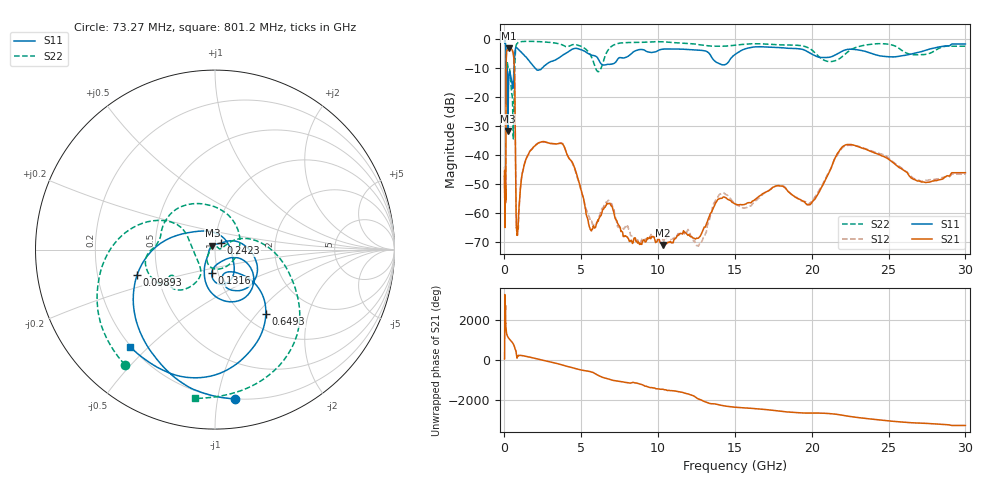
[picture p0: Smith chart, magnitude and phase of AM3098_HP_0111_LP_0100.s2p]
! Date/Time: Thu, Feb 28, 2019 8:38 AM
! Network Analyzer: Agilent Technologies E8364B Rev: A.07.50.67
! Sweep from 0.010 to 30.000 GHz, 1601 Points, Sweep Type: LOG
! Power Supply: 5.022 V, 0.002 A
# Hz S DB R 50
!freq MagS11 AngS11 MagS21 AngS21 MagS12 AngS12 MagS22 AngS22
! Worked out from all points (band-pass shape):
!   1601 points, 10 MHz to 30 GHz, reference 50 ohm
!   highest |S21| = -3.07 dB at 266.5 MHz (marker M1); lowest = -71.0 dB at 10.33 GHz (marker M2)
!   |S21| within 3 dB of the highest: 120.9 MHz to 602.1 MHz (481.2 MHz wide, 133 % of centre)
!   lowest |S11| = -31.6 dB at 232.8 MHz (marker M3), VSWR 1.05, Z = 48.5 + j2.13 ohm
!   |S11| at or under -10 dB: 102.2 MHz to 619.4 MHz (517.2 MHz wide, 143 % of centre); 2.012 GHz to 2.43 GHz (418.4 MHz wide, 18.8 % of centre)
!   |S22| runs from -34.3 to -0.5 dB; largest |S21 - S12| = 0.0098
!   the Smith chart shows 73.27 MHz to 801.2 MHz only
!   S11 on the Smith chart (normalised r, x): 73.27 MHz: 0.20, -1.12; 98.93 MHz: 0.38, -0.13; 131.6 MHz: 0.93, -0.25; 242.3 MHz: 1.07, +0.08; 649.3 MHz: 1.23, -1.12; 801.2 MHz: 0.20, -0.44
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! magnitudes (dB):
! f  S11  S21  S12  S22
! 10 MHz  -0.3  -47.1  -44.4  -0.5
! 38.04 MHz  -0.4  -59.5  -59.7  -0.8
! 73.27 MHz  -1.5  -54.0  -53.6  -1.8
! 86.86 MHz  -2.9  -51.9  -52.2  -3.0
! 98.93 MHz  -6.8  -26.3  -26.0  -7.8
! 131.6 MHz  -17.5  -4.9  -4.9  -10.3
! 144.7 MHz  -20.2  -4.1  -4.1  -11.2
! 184.9 MHz  -10.7  -3.7  -3.7  -8.0
! 232.8 MHz  -31.6  -3.2  -3.2  -9.7
! 242.3 MHz  -26.3  -3.2  -3.1  -9.8
! 266.5 MHz  -15.7  -3.1  -3.0  -10.1
! 550.5 MHz  -16.9  -4.4  -4.3  -30.3
! 649.3 MHz  -6.8  -10.8  -10.7  -14.3
! 801.2 MHz  -2.9  -65.9  -65.8  -1.5
! 2.084 GHz  -10.4  -36.3  -36.2  -0.7
! 3.798 GHz  -5.4  -36.2  -36.0  -2.0
! 5.584 GHz  -5.2  -65.6  -62.6  -5.2
! 7.926 GHz  -6.1  -68.0  -65.0  -1.1
! 10.33 GHz  -3.3  -71.0  -69.3  -0.8
! 19.8 GHz  -4.5  -57.1  -56.8  -3.0
! 22.56 GHz  -3.4  -36.3  -36.6  -3.5
! 30 GHz  -1.6  -46.0  -46.6  -2.3
